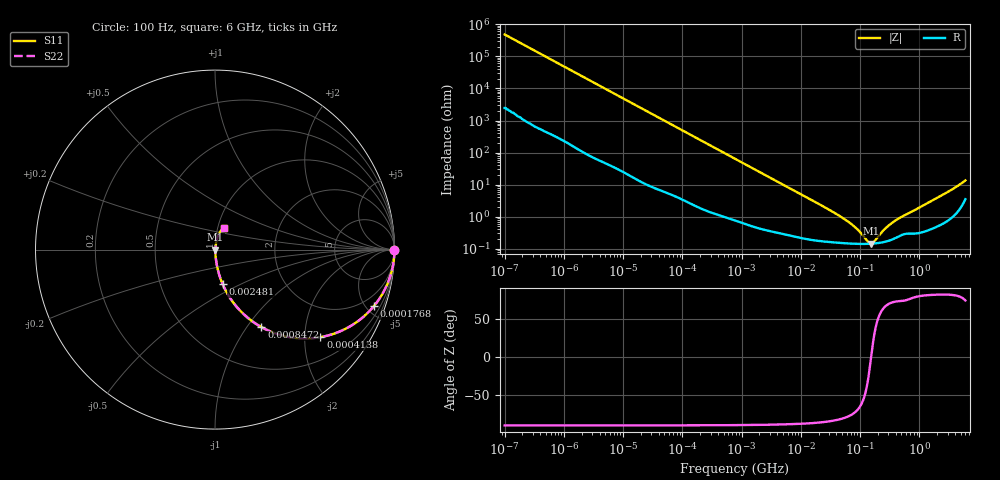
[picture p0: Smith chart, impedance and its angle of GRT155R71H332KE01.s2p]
!Murata Part Number: GRT155R71H332KE01
!These Parameters are Measured in Series Mode Connection
!Data Generated on Jun 19, 2026
!  o--ll--o
!Port1  Port2
!  o------o
!Operation Temp=25[degC], DC Bias Voltage=0[V]
!Freq. Start=100[Hz] Stop=6[GHz] 401[Steps]
# Hz S RI R 50
!Freq.(Hz) S11(Real) S11(Imag) S21(Real) S21(Imag) S12(Real) S12(Imag) S22(Real) S22(Imag)
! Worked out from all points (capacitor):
!   401 points, 100 Hz to 6 GHz, reference 50 ohm
!   read as one part in series: C = 3.3 nF near 109 Hz
!   lowest |Z| = 144 mohm at 152.6 MHz (marker M1)
!   series resonance near 153.5 MHz, so ESL is about 330 pH
!   S11 on the Smith chart (normalised r, x): 100 Hz: open; 176.8 kHz: 1.04, -5.58; 413.8 kHz: 1.02, -2.39; 847.2 kHz: 1.01, -1.17; 2.481 MHz: 1.01, -0.40; 6 GHz: 1.07, +0.26
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100  1 -0.000208  1.1e-06 0.000208  1.1e-06 0.000208  1 -0.000208
2008  1 -0.00413  3.56e-05 0.00413  3.56e-05 0.00413  1 -0.00413
40335  0.9928 -0.0817  0.00719 0.0817  0.00719 0.0817  0.9928 -0.0817
98762  0.96 -0.1925  0.04 0.1925  0.04 0.1925  0.96 -0.1925
176758  0.8843 -0.3162  0.1157 0.3162  0.1157 0.3162  0.8843 -0.3162
264476  0.7752 -0.4135  0.2248 0.4135  0.2248 0.4135  0.7752 -0.4135
413847  0.5874 -0.4876  0.4126 0.4876  0.4126 0.4876  0.5874 -0.4876
774597  0.2934 -0.4494  0.7066 0.4494  0.7066 0.4494  0.2934 -0.4494
847162  0.2585 -0.4316  0.7415 0.4316  0.7415 0.4316  0.2585 -0.4316
1386327  0.118 -0.3154  0.882 0.3154  0.882 0.3154  0.118 -0.3154
2481164  0.0424 -0.1922  0.9576 0.1922  0.9576 0.1922  0.0424 -0.1922
5554849  0.0108 -0.0894  0.9892 0.0894  0.9892 0.0894  0.0108 -0.0894
1.555665e7  0.00292 -0.0323  0.9971 0.0323  0.9971 0.0323  0.00292 -0.0323
6.233367e7  0.00151 -0.00693  0.9985 0.00693  0.9985 0.00693  0.00151 -0.00693
9.326766e7  0.00143 -0.00352  0.9986 0.00352  0.9986 0.00352  0.00143 -0.00352
1.334425e8  0.00142 -0.000955  0.9986 0.000955  0.9986 0.000955  0.00142 -0.000955
1.526266e8  0.00144 -3.89e-05  0.9986 3.89e-05  0.9986 3.89e-05  0.00144 -3.89e-05
1.745687e8  0.00147 0.000877  0.9985 -0.000877  0.9985 -0.000877  0.00147 0.000877
3.124326e8  0.00183 0.00522  0.9982 -0.00522  0.9982 -0.00522  0.00183 0.00522
4.674818e8  0.00259 0.00884  0.9974 -0.00884  0.9974 -0.00884  0.00259 0.00884
1.95892e9  0.0062 0.0372  0.9938 -0.0372  0.9938 -0.0372  0.0062 0.0372
6e9  0.0492 0.1205  0.9508 -0.1205  0.9508 -0.1205  0.0492 0.1205
